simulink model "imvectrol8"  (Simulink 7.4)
settings: Solver=ode45  StartTime=0.0  StopTime=2.5  MaxStep=1e-4  RelTol=1e-3  AbsTol=1e-3
InitFcn:
  | param8
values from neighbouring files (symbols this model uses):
  Bm = 0.10    (= 0.1)    [IMabc2.m]    (also in imabcparam.m = 0.01; IMabcrun0.m = 0.01; IMabcrun1.m = 0.001; IMcur0.m = 1e-06)
  J = 0.02    [imabcparam.m]    (also in IMabcrun0.m; IMabcrun1.m; imdefSIvec1.m = 0.03)
  Lm = eval(get(hLm,'String'))    [im3d.m]    (also in IMabc2.m = 4.5; imabcparam.m = 0.0847; IMabcrun0.m = 0.0847; IMabcrun1.m = 0.0847)
  Lr = Lrl+Lm    (= 4.6)    [IMabc2.m]    (also in IMabcf0.m = Lrl+Lm1; IMabcf1.m = Lrl+Lm1; imabcparam.m = 0.0589666666667; IMcur0.m)
  p = cos(beta-alpha)    [abcRwdg.m]    (also in alternator.m = 0:pi/20:2*pi; altwdgs.m = 0:pi/20:2*pi; brushlessdcB.m = 0:pi/100:2*pi; brushlessdcnew.m = 0:pi/100:2*pi)
undefined symbols (not defined in the file or in its folder): ktune, taur

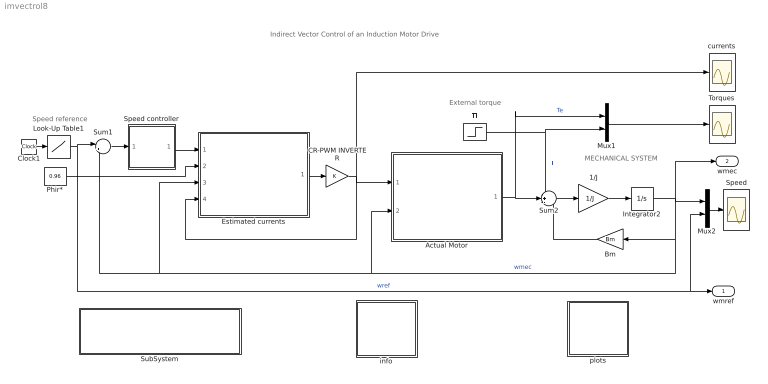
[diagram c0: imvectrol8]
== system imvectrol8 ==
  note: Indirect Vector Control of an Induction Motor Drive
  note: Speed reference
  note: External torque
  note: MECHANICAL SYSTEM
  1/J : Gain  Gain=1/J  ParameterDataType=sfix(16)  ParameterScaling=2^0  OutDataType=sfix(16)  OutScaling=2^0
  Actual Motor : Subsystem
  Bm : Gain  Gain=Bm  ParameterDataType=sfix(16)  ParameterScaling=2^0  OutDataType=sfix(16)  OutScaling=2^0
  CR-PWM INVERTER : Gain  ParameterDataType=sfix(16)  ParameterScaling=2^0  OutDataType=sfix(16)  OutScaling=2^0
  Clock1 : Clock
  Estimated currents : Subsystem
  Integrator2 : Integrator  InitialCondition=120
  Look-Up Table1 : Lookup  InputValues="[0  .2 .201 1.5  1.501 2]"  Table=[120 120 180 180 60 60 ]  OutDataType=sfix(16)  OutScaling=2^0
  Mux1 : Mux  Inputs=2
  Mux2 : Mux  Inputs=2
  Phir* : Constant  Value=0.96  OutDataType=sfix(16)  OutScaling=2^0
  Speed : Scope
  Speed controller : Subsystem  mask(PI controller){Kp=100, Ki=2500, Tlim=350, Ts=0}
      mask prompts: Kp "Proportional gain (Kp)"; Ki "Integral gain (Ki)"; Tlim "Torque limit (N.m)"; Ts "Sampling time (s)"
      mask help: Proportional-Integral Speed Controller
  SubSystem : Subsystem
  Sum1 : Sum  Inputs=|+-  OutDataType=sfix(16)  OutScaling=2^0
  Sum2 : Sum  Inputs=-+-  OutDataType=sfix(16)  OutScaling=2^0
  Tl : Step  After=200  SampleTime=0
  Torques : Scope
  currents : Scope
  info : Subsystem
  plots : Subsystem
  wmref : Outport
  wmec : Outport  Port=2
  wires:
  Sum2/1 -> 1/J/1
  1/J/1 -> Integrator2/1
  Integrator2/1 -> Bm/1, Actual Motor/2(wmech), Sum1/2, Estimated currents/3(wmec), Mux2/1, wmec/1  "wmec"
  Bm/1 -> Sum2/3
  Sum1/1 -> Speed controller/1(we)
  Mux1/1 -> Torques/1
  Tl/1 -> Mux1/2, Sum2/1  "Tl"
  Estimated currents/1(iabc*) -> CR-PWM INVERTER/1
  Speed controller/1(Te*) -> Estimated currents/1(Te*)
  Phir*/1 -> Estimated currents/2(phir*)
  Clock1/1 -> Look-Up Table1/1
  Mux2/1 -> Speed/1
  Look-Up Table1/1 -> Sum1/1, Mux2/2, wmref/1  "wref"
  CR-PWM INVERTER/1 -> Actual Motor/1(Iabc), Estimated currents/4(iabc), currents/1
  Actual Motor/1(Te) -> Sum2/2, Mux1/1  "Te"

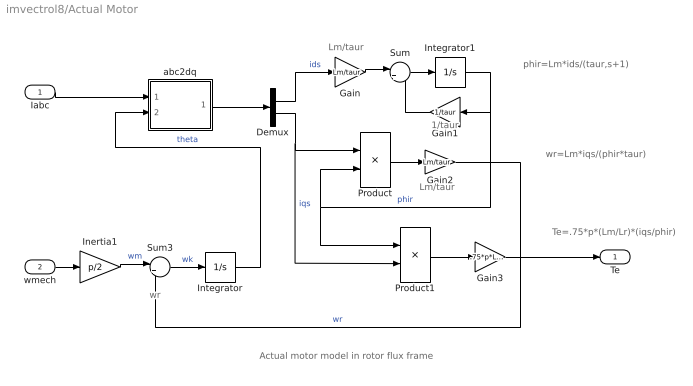
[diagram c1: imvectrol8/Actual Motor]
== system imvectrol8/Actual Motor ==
  note: Lm/taur
  note: 1/taur
  note: Lm/taur
  note: Te=.75*p*(Lm/Lr)*(iqs/phir)
  note: Actual motor model in rotor flux frame
  note: wr
  note: wr=Lm*iqs/(phir*taur)
  note: phir=Lm*ids/(taur,s+1)
  Iabc : Inport  OutDataType=sfix(16)  OutScaling=2^0
  wmech : Inport  Port=2  OutDataType=sfix(16)  OutScaling=2^0
  Demux : Demux  Outputs=2
  Gain : Gain  Gain=Lm/taur  ParameterDataType=sfix(16)  ParameterScaling=2^0  OutDataType=sfix(16)  OutScaling=2^0
  Gain1 : Gain  Gain=1/taur  ParameterDataType=sfix(16)  ParameterScaling=2^0  OutDataType=sfix(16)  OutScaling=2^0
  Gain2 : Gain  Gain=Lm/taur  ParameterDataType=sfix(16)  ParameterScaling=2^0  OutDataType=sfix(16)  OutScaling=2^0
  Gain3 : Gain  Gain=.75*p*Lm/Lr  ParameterDataType=sfix(16)  ParameterScaling=2^0  OutDataType=sfix(16)  OutScaling=2^0
  Inertia1 : Gain  Gain=p/2  ParameterDataType=sfix(16)  ParameterScaling=2^0  OutDataType=sfix(16)  OutScaling=2^0
  Integrator : Integrator
  Integrator1 : Integrator  InitialCondition=1
  Product : Product  Inputs=*/  OutDataType=sfix(16)  OutScaling=2^0
  Product1 : Product  OutDataType=sfix(16)  OutScaling=2^0
  Sum : Sum  Inputs=|+-  OutDataType=sfix(16)  OutScaling=2^0
  Sum3 : Sum  Inputs=|++  OutDataType=sfix(16)  OutScaling=2^0
  abc2dq : Subsystem
  Te : Outport
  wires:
  Demux/1 -> Gain/1  "ids"
  Sum/1 -> Integrator1/1
  Integrator1/1 -> Gain1/1, Product/2, Product1/1  "phir"
  Demux/2 -> Product/1, Product1/2  "iqs"
  Product/1 -> Gain2/1
  Product1/1 -> Gain3/1
  Sum3/1 -> Integrator/1  "wk"
  Inertia1/1 -> Sum3/1  "wm"
  Gain2/1 -> Sum3/2  "wr"
  Integrator/1 -> abc2dq/2(theta)  "theta"
  wmech/1 -> Inertia1/1
  Gain3/1 -> Te/1
  Iabc/1 -> abc2dq/1(iabc)
  abc2dq/1(idq) -> Demux/1
  Gain/1 -> Sum/1
  Gain1/1 -> Sum/2

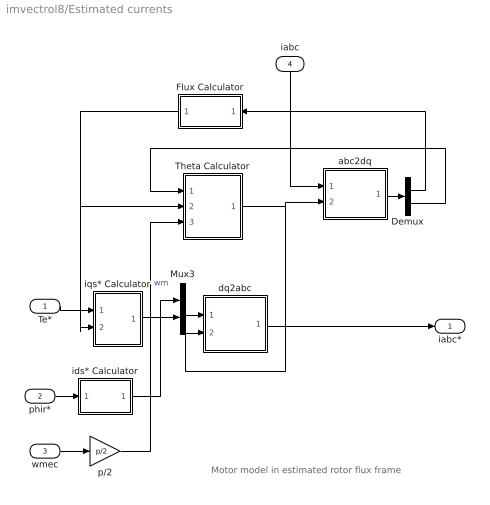
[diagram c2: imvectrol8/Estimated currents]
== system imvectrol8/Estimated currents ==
  note: Motor model in estimated rotor flux frame
  Te* : Inport  OutDataType=sfix(16)  OutScaling=2^0
  phir* : Inport  Port=2  OutDataType=sfix(16)  OutScaling=2^0
  wmec : Inport  Port=3  OutDataType=sfix(16)  OutScaling=2^0
  iabc : Inport  Port=4  OutDataType=sfix(16)  OutScaling=2^0
  Demux : Demux  Outputs=2
  Flux Calculator : Subsystem
  Mux3 : Mux  Inputs=2
  Theta Calculator : Subsystem
  abc2dq : Subsystem
  dq2abc : Subsystem
  ids* Calculator : Subsystem
  iqs* Calculator : Subsystem
  p/2 : Gain  Gain=p/2  ParameterDataType=sfix(16)  ParameterScaling=2^0  OutDataType=sfix(16)  OutScaling=2^0
  iabc* : Outport
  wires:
  iqs* Calculator/1(Iq*) -> Mux3/2
  ids* Calculator/1(Id*) -> Mux3/1
  Flux Calculator/1(Phir) -> Theta Calculator/2(Phir), iqs* Calculator/2(Phir)
  Mux3/1 -> dq2abc/1(idq*)
  Theta Calculator/1(theta*) -> dq2abc/2(theta*), abc2dq/2(theta*)
  Demux/1 -> Flux Calculator/1(Id)
  Demux/2 -> Theta Calculator/1(Iq)
  abc2dq/1(idq) -> Demux/1
  p/2/1 -> Theta Calculator/3(wm)  "wm"
  dq2abc/1(iabc^) -> iabc*/1
  Te*/1 -> iqs* Calculator/1(Te*)
  phir*/1 -> ids* Calculator/1(Phir*)
  wmec/1 -> p/2/1
  iabc/1 -> abc2dq/1(iabc)

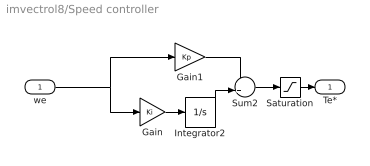
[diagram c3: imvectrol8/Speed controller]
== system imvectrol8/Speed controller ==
  we : Inport  OutDataType=sfix(16)  OutScaling=2^0
  Gain : Gain  Gain=Ki  ParameterDataType=sfix(16)  ParameterScaling=2^0  OutDataType=sfix(16)  OutScaling=2^0
  Gain1 : Gain  Gain=Kp  ParameterDataType=sfix(16)  ParameterScaling=2^0  OutDataType=sfix(16)  OutScaling=2^0
  Integrator2 : Integrator  LimitOutput=on  UpperSaturationLimit=Tlim  LowerSaturationLimit=-Tlim
  Saturation : Saturate  UpperLimit=Tlim  LowerLimit=-Tlim
  Sum2 : Sum  OutDataType=sfix(16)  OutScaling=2^0
  Te* : Outport  InitialOutput=0
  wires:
  Gain1/1 -> Sum2/1
  Gain/1 -> Integrator2/1
  Saturation/1 -> Te*/1
  we/1 -> Gain/1, Gain1/1
  Sum2/1 -> Saturation/1
  Integrator2/1 -> Sum2/2

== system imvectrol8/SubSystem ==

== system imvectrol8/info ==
  note: A three-phase induction motor rated at 50hp, 460V,4pole,60Hz is modeled in the rotor flux reference frame.The speed loop utilizes a PI controller to produce the quadrature-axis currents iq* which serves as the torque command. The derived direct-axis current id* serves as the rotor flux command. These currents are then transformed via the block into the currrent references ia*, ib*, and ic* fed into the current-regulated PWM inverter. Rotor flux field orientation is obtained in the block. The parameters are entered via a callback in Model Properties and a specific steady-state operation at wref=120rad/s and Tl=0 is then established. Examine the transient response due to step changes in the command speed wref and load torque Tl. Repeat the simulation for a detuned condition when the estimated value of the rotor time constant Taur appearing in the differs from the actual value used for the motor parameters (ktune=1.0 for perfect tuning).
  note: (adapted from Power System Blockset case study)
  note: Indirect Vector Control of an Induction Motor Drive Current-regulated PPU

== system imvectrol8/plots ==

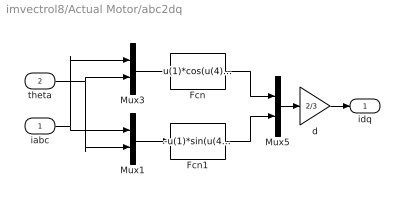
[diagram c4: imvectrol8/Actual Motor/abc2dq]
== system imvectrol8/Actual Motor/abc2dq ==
  iabc : Inport  OutDataType=sfix(16)  OutScaling=2^0
  theta : Inport  Port=2  OutDataType=sfix(16)  OutScaling=2^0
  Fcn : Fcn  Expr=u(1)*cos(u(4))+u(2)*cos(u(4)-2*pi/3)+u(3)*cos(u(4)+2*pi/3)
  Fcn1 : Fcn  Expr=-u(1)*sin(u(4))-u(2)*sin(u(4)-2*pi/3)-u(3)*sin(u(4)+2*pi/3)
  Mux1 : Mux  Inputs=2
  Mux3 : Mux  Inputs=2
  Mux5 : Mux  Inputs=2
  d : Gain  Gain=2/3  ParameterDataType=sfix(16)  ParameterScaling=2^0  OutDataType=sfix(16)  OutScaling=2^0
  idq : Outport
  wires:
  Mux3/1 -> Fcn/1
  Fcn/1 -> Mux5/1
  Mux5/1 -> d/1
  Mux1/1 -> Fcn1/1
  Fcn1/1 -> Mux5/2
  iabc/1 -> Mux1/1, Mux3/1
  theta/1 -> Mux3/2, Mux1/2
  d/1 -> idq/1

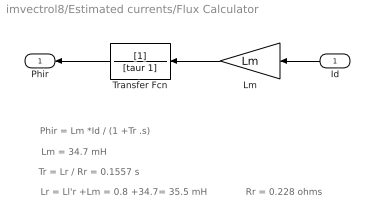
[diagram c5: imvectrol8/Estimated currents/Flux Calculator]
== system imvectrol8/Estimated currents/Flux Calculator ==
  note: Phir = Lm *Id / (1 +Tr .s)
  note: Lm = 34.7 mH
  note: Lr = Ll'r +Lm = 0.8 +34.7= 35.5 mH
  note: Tr = Lr / Rr = 0.1557 s
  note: Rr = 0.228 ohms
  Id : Inport  OutDataType=sfix(16)  OutScaling=2^0
  Lm : Gain  Gain=Lm  ParameterDataType=sfix(16)  ParameterScaling=2^0  OutDataType=sfix(16)  OutScaling=2^0
  Transfer Fcn : TransferFcn  Denominator=[taur 1]
  Phir : Outport
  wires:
  Transfer Fcn/1 -> Phir/1
  Id/1 -> Lm/1
  Lm/1 -> Transfer Fcn/1

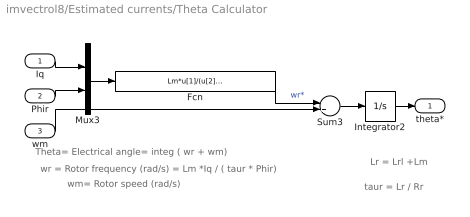
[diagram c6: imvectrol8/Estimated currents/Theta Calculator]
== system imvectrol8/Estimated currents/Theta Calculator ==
  note: Theta= Electrical angle= integ ( wr + wm)
  note: wr = Rotor frequency (rad/s) = Lm *Iq / ( taur * Phir)
  note: Lr = Lrl +Lm
  note: wm= Rotor speed (rad/s)
  note: taur = Lr / Rr
  Iq : Inport  OutDataType=sfix(16)  OutScaling=2^0
  Phir : Inport  Port=2  OutDataType=sfix(16)  OutScaling=2^0
  wm : Inport  Port=3  OutDataType=sfix(16)  OutScaling=2^0
  Fcn : Fcn  Expr=Lm*u[1]/(u[2]*taur*ktune+1e-3)
  Integrator2 : Integrator
  Mux3 : Mux  Inputs=2
  Sum3 : Sum  OutDataType=sfix(16)  OutScaling=2^0
  theta* : Outport  InitialOutput=0
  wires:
  Integrator2/1 -> theta*/1
  wm/1 -> Sum3/2
  Fcn/1 -> Sum3/1  "wr*"
  Phir/1 -> Mux3/2
  Iq/1 -> Mux3/1
  Mux3/1 -> Fcn/1
  Sum3/1 -> Integrator2/1

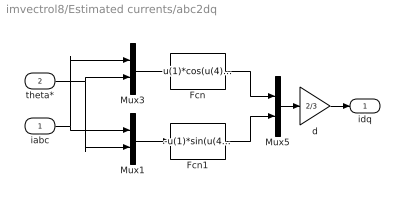
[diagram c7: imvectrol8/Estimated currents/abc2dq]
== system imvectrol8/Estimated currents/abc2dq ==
  iabc : Inport  OutDataType=sfix(16)  OutScaling=2^0
  theta* : Inport  Port=2  OutDataType=sfix(16)  OutScaling=2^0
  Fcn : Fcn  Expr=u(1)*cos(u(4))+u(2)*cos(u(4)-2*pi/3)+u(3)*cos(u(4)+2*pi/3)
  Fcn1 : Fcn  Expr=-u(1)*sin(u(4))-u(2)*sin(u(4)-2*pi/3)-u(3)*sin(u(4)+2*pi/3)
  Mux1 : Mux  Inputs=2
  Mux3 : Mux  Inputs=2
  Mux5 : Mux  Inputs=2
  d : Gain  Gain=2/3  ParameterDataType=sfix(16)  ParameterScaling=2^0  OutDataType=sfix(16)  OutScaling=2^0
  idq : Outport
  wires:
  Mux3/1 -> Fcn/1
  Fcn/1 -> Mux5/1
  Mux5/1 -> d/1
  Mux1/1 -> Fcn1/1
  Fcn1/1 -> Mux5/2
  iabc/1 -> Mux1/1, Mux3/1
  theta*/1 -> Mux3/2, Mux1/2
  d/1 -> idq/1

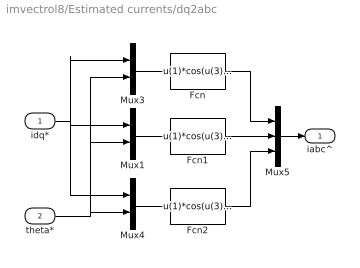
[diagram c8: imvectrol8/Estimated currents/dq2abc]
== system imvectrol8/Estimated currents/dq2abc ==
  idq* : Inport  OutDataType=sfix(16)  OutScaling=2^0
  theta* : Inport  Port=2  OutDataType=sfix(16)  OutScaling=2^0
  Fcn : Fcn  Expr=u(1)*cos(u(3))-u(2)*sin(u(3))
  Fcn1 : Fcn  Expr=u(1)*cos(u(3)-2*pi/3)-u(2)*sin(u(3)-2*pi/3)
  Fcn2 : Fcn  Expr=u(1)*cos(u(3)+2*pi/3)-u(2)*sin(u(3)+2*pi/3)
  Mux1 : Mux  Inputs=2
  Mux3 : Mux  Inputs=2
  Mux4 : Mux  Inputs=2
  Mux5 : Mux  Inputs=3
  iabc^ : Outport
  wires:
  Mux3/1 -> Fcn/1
  Mux4/1 -> Fcn2/1
  idq*/1 -> Mux3/1, Mux4/1, Mux1/1
  Fcn/1 -> Mux5/1
  Mux5/1 -> iabc^/1
  Mux1/1 -> Fcn1/1
  Fcn1/1 -> Mux5/2
  Fcn2/1 -> Mux5/3
  theta*/1 -> Mux4/2, Mux3/2, Mux1/2

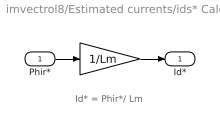
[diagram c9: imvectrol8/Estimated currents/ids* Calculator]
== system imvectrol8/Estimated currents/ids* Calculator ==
  note: Id* = Phir*/ Lm
  Phir* : Inport  OutDataType=sfix(16)  OutScaling=2^0
  " " : Gain  Gain=1/Lm  ParameterDataType=sfix(16)  ParameterScaling=2^0  OutDataType=sfix(16)  OutScaling=2^0
  Id* : Outport
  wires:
  " "/1 -> Id*/1
  Phir*/1 -> " "/1

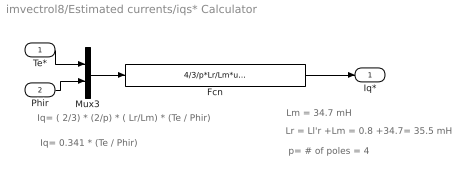
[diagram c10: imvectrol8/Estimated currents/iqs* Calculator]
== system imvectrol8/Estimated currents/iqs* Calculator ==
  note: Iq= ( 2/3) * (2/p) * ( Lr/Lm) * (Te / Phir)
  note: Lm = 34.7 mH
  note: Lr = Ll'r +Lm = 0.8 +34.7= 35.5 mH
  note: p= # of poles = 4
  note: Iq= 0.341 * (Te / Phir)
  Te* : Inport  OutDataType=sfix(16)  OutScaling=2^0
  Phir : Inport  Port=2  OutDataType=sfix(16)  OutScaling=2^0
  Fcn : Fcn  Expr=4/3/p*Lr/Lm*u[1]/(u[2]+1e-3)
  Mux3 : Mux  Inputs=2
  Iq* : Outport  InitialOutput=0
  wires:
  Fcn/1 -> Iq*/1
  Te*/1 -> Mux3/1
  Mux3/1 -> Fcn/1
  Phir/1 -> Mux3/2
